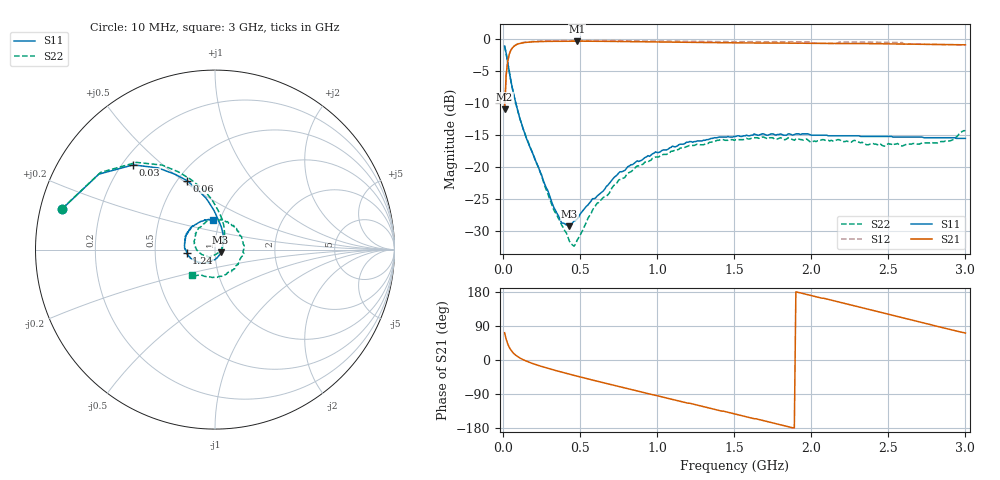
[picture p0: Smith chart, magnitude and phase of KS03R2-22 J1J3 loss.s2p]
! "!Agilent Technologies,E5071B,MY42403564,A.08.11"
!Date: Wed Apr 07 12:16:23 2010
!Data & Calibration Information:
!Freq	S11:SOLT2(ON)	S21:SOLT2(ON)	S12:SOLT2(ON)	S22:SOLT2(ON)
# Hz S dB R 50
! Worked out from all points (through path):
!   300 points, 10 MHz to 3 GHz, reference 50 ohm
!   highest |S21| = -0.35 dB at 480 MHz (marker M1); lowest = -11.0 dB at 10 MHz (marker M2)
!   group delay of S21, straight-line fit = 278 ps
!   lowest |S11| = -29.2 dB at 430 MHz (marker M3), VSWR 1.07, Z = 53.2 - j1.57 ohm
!   |S11| at or under -10 dB: 82.55 MHz to end of sweep
!   |S22| runs from -32.3 to -1.1 dB; largest |S21 - S12| = 0.029
!   S11 on the Smith chart (normalised r, x): 10 MHz: 0.06, +0.13; 30 MHz: 0.24, +0.40; 60 MHz: 0.56, +0.52; 1.24 GHz: 0.73, -0.02; 3 GHz: 0.93, +0.32
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1e7  -1.11 165.0  -11.00 72.0  -11.00 72.1  -1.09 165.0
2e7  -2.25 147.0  -5.67 55.1  -5.65 55.2  -2.28 146.0
3e7  -3.66 134.0  -3.51 42.7  -3.49 42.7  -3.69 132.0
6e7  -7.65 112.0  -1.41 21.4  -1.37 21.3  -7.68 109.0
1e8  -11.60 97.1  -0.77 7.6  -0.72 7.7  -11.60 91.7
1.7e8  -16.60 79.3  -0.49 -6.0  -0.44 -6.0  -16.50 71.7
3.3e8  -26.30 28.5  -0.37 -26.4  -0.29 -26.4  -26.70 22.8
3.8e8  -28.70 5.5  -0.35 -31.9  -0.26 -31.9  -29.00 -0.8
4.3e8  -29.20 -25.1  -0.35 -37.3  -0.26 -37.3  -31.50 -32.7
4.8e8  -28.10 -55.1  -0.35 -42.6  -0.25 -42.5  -31.40 -76.1
5.1e8  -27.00 -69.6  -0.35 -45.6  -0.25 -45.7  -30.10 -97.7
6.1e8  -24.50 -101.0  -0.37 -55.9  -0.26 -55.8  -25.60 -127.0
7.5e8  -20.90 -124.0  -0.40 -69.9  -0.28 -69.9  -22.00 -160.0
1.01e9  -17.70 -154.0  -0.48 -95.3  -0.32 -95.3  -18.40 161.0
1.24e9  -16.00 -174.0  -0.55 -117.0  -0.38 -117.0  -16.60 129.0
1.51e9  -15.20 164.0  -0.62 -143.0  -0.43 -143.0  -15.70 93.9
1.76e9  -14.90 147.0  -0.64 -167.0  -0.42 -167.0  -15.60 63.2
2.01e9  -15.00 132.0  -0.68 169.0  -0.68 169.0  -16.00 31.4
2.24e9  -15.10 120.0  -0.71 147.0  -0.47 147.0  -16.00 -1.4
2.51e9  -15.20 108.0  -0.78 120.0  -0.54 120.0  -16.40 -45.1
2.75e9  -15.40 101.0  -0.85 95.8  -0.85 95.9  -16.20 -90.4
3e9  -15.50 93.6  -0.92 71.1  -0.92 71.1  -14.30 -132.0
